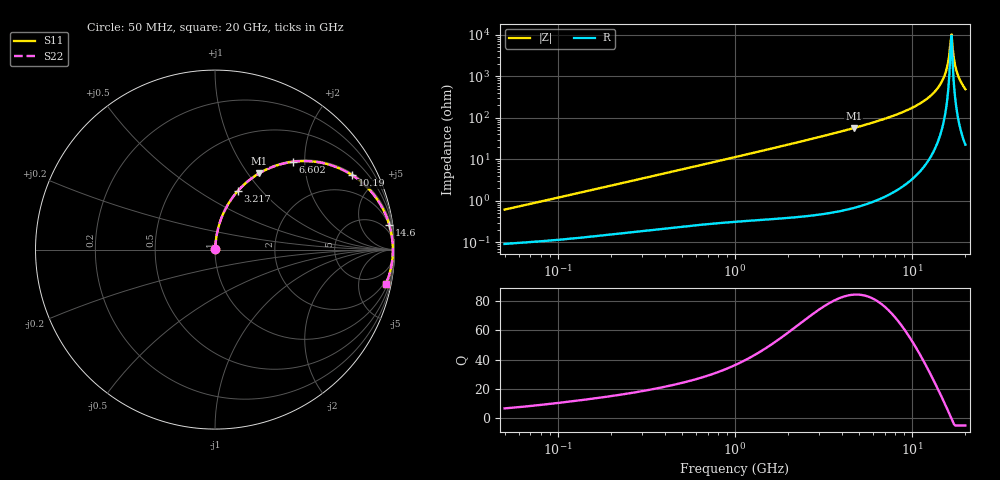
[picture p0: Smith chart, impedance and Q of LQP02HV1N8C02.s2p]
!Murata Part Number: LQP02HV1N8C02
!These Parameters are Measured in Series Mode Connection
!  o--[Z]--o
!Port1  Port2
!  o-------o
!Freq. Start=50[MHz] Stop=20[GHz], 401[Steps]
# Hz S RI R 50
!Freq.(Hz) S11(Real) S11(Imag) S21(Real) S21(Imag) S12(Real) S12(Imag) S22(Real) S22(Imag)
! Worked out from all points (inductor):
!   401 points, 50 MHz to 20 GHz, reference 50 ohm
!   read as one part in series: L = 1.92 nH near 51.52 MHz
!   highest Q = 84.3 at 4.678 GHz (marker M1), where L = 1.93 nH
!   self-resonance near 16.46 GHz
!   S11 on the Smith chart (normalised r, x): 50 MHz: 1.00, +0.01; 3.217 GHz: 1.01, +0.75; 6.602 GHz: 1.02, +1.75; 10.19 GHz: 1.07, +3.64; 14.6 GHz: 2, +14; 20 GHz: 1.45, -9.82
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5e7  0.000951 0.00608  0.999 -0.00608  0.999 -0.00608  0.000951 0.00608
1.364002e8  0.00156 0.016  0.9984 -0.016  0.9984 -0.016  0.00156 0.016
3.721004e8  0.00388 0.0424  0.9961 -0.0424  0.9961 -0.0424  0.00388 0.0424
1e9  0.0156 0.1109  0.9844 -0.1109  0.9844 -0.1109  0.0156 0.1109
2.728004e9  0.0928 0.2832  0.9072 -0.2832  0.9072 -0.2832  0.0928 0.2832
3.216634e9  0.1257 0.325  0.8743 -0.325  0.8743 -0.325  0.1257 0.325
4.677679e9  0.2461 0.4249  0.7539 -0.4249  0.7539 -0.4249  0.2461 0.4249
6.601595e9  0.4343 0.4893  0.5657 -0.4893  0.5657 -0.4893  0.4343 0.4893
7.442007e9  0.5186 0.4929  0.4814 -0.4929  0.4814 -0.4929  0.5186 0.4929
1.019291e10  0.7636 0.4152  0.2364 -0.4152  0.2364 -0.4152  0.7636 0.4152
1.276073e10  0.9148 0.2627  0.0852 -0.2627  0.0852 -0.2627  0.9148 0.2627
1.460232e10  0.9715 0.1367  0.0285 -0.1367  0.0285 -0.1367  0.9715 0.1367
1.550395e10  0.9851 0.0754  0.0149 -0.0754  0.0149 -0.0754  0.9851 0.0754
1.573793e10  0.9873 0.0597  0.0127 -0.0597  0.0127 -0.0597  0.9873 0.0597
1.621653e10  0.9901 0.0282  0.00987 -0.0282  0.00987 -0.0282  0.9901 0.0282
1.646126e10  0.9908 0.0124  0.00919 -0.0124  0.00919 -0.0124  0.9908 0.0124
1.670968e10  0.991 -0.00349  0.00902 0.00349  0.00902 0.00349  0.991 -0.00349
1.696185e10  0.9906 -0.0193  0.00936 0.0193  0.00936 0.0193  0.9906 -0.0193
1.774144e10  0.9866 -0.0668  0.0134 0.0668  0.0134 0.0668  0.9866 -0.0668
1.828096e10  0.9813 -0.0981  0.0187 0.0981  0.0187 0.0981  0.9813 -0.0981
1.912117e10  0.9696 -0.1445  0.0304 0.1445  0.0304 0.1445  0.9696 -0.1445
2e10  0.9521 -0.1917  0.0479 0.1917  0.0479 0.1917  0.9521 -0.1917
